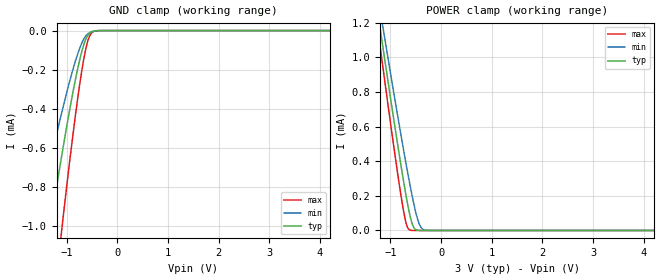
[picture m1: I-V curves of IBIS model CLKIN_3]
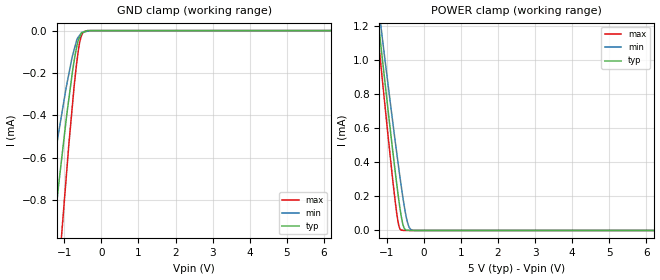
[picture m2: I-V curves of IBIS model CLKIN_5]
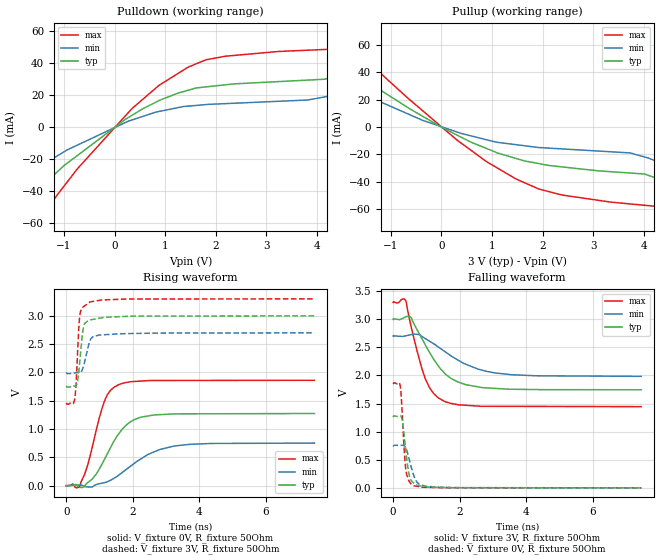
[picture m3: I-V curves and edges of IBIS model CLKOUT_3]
|Texas Instruments Incorporated
|Two 1-Bit, 10MHz, 2nd - Order Delta-Sigma Modulators
| Marketing part#   Digital Voltage Range   Package-type   #pins
|ADS1205IRGER   2.7V to 5.5V   QFN   24
|ADS1205IRGET   2.7V to 5.5V   QFN   24
|ADS1209SPW   2.7V to 5.5V   TSSOP   24
|ADS1209SPWR   2.7V to 5.5V   TSSOP   24
[IBIS Ver]   4.0
[File name]   ads1205_9.ibs
[File Rev]   1.0
[Date]   02/23/2010
[Source]   Texas Instruments Incorporated.
   Analog-eLab, HPA
   12500 TI Blvd
   Dallas, TX -75243
   For Support e-mail: elab_ibis@list.ti.com
[Notes]   Revision History:
   1.0: 02/23/2010
   - Initial version of the model
   - Initial Model generated from simulations in TIspiceD
   - Model names with a trailing _3 contains the model for
   3V [2.7V and 3.3V]. Model names with trailing _5 contains
   the model for 5V [4.5V and 5.5V] operation.
   - Model not matched to measurements
   - C_comp: Ignore warnings related to min and max values of
   ccomp. The device process of these products is CMOS. The
   ccomp values are based on PVT variations as seen in
   simulations
[Disclaimer]
 This product is designed as an aid for customers of Texas Instruments.
 No warranties, either expressed or implied, with respect to this third
 party software [if any] or with respect to its fitness for any
 particular purpose is claimed by Texas Instruments or the author. The
 software [if any] is provided solely on an "as is" basis. The entire
 risk as to its quality and performance is with the customer
[Copyright] [C] Copyright 2010 Texas Instruments Incorporated.
   All rights reserved.
|   ADS1205
[Component]   ADS1205rge
[Manufacturer] TI   |QFN package, 24-pin
[Package]
|variable   typ   min   max
R_pkg   0.041250   0.000780   0.051560
L_pkg   0.989262nH   0.176530nH   1.226320nH
C_pkg   0.170271pF   0.099550pF   0.190160pF
[Pin] signal_name  model_name  R_pin  L_pin C_pin
1   REFINB   TERM   0.04895  1.17050nH  0.16737pF
2   AGND   TERM   0.04084  0.96823nH  0.17417pF
3   AVDD   TERM   0.03902  0.92564nH  0.17135pF
4   AVDD   TERM   0.03955  0.93760nH  0.17281pF
5   AGND   TERM   0.04334  1.02645nH  0.18033pF
6   CLKSEL   CLKSEL   0.04571  1.09072nH  0.16450pF
7   CLKIN   CLKIN   0.04780  1.14015nH  0.16895pF
8   BVDD   POWER   0.04468  1.05593nH  0.18370pF
9   BGND   GND   0.04453  1.04910nH  0.18273pF
10   CLKOUT   CLKOUT   0.04778  1.12594nH  0.18715pF
11   OUTB   OUTB   0.05004  1.18148nH  0.19016pF
12   OUTA   OUTA   0.05156  1.22632nH  0.17289pF
13   AGND   TERM   0.04529  1.07336nH  0.16265pF
14   REFOUT   TERM   0.04455  1.04803nH  0.18209pF
15   AVDD   TERM   0.03980  0.93443nH  0.17351pF
16   AVDD   TERM   0.03902  0.91648nH  0.17120pF
17   AGND   TERM   0.04084  0.95994nH  0.17392pF
18   REFINA   TERM   0.04895  1.16087nH  0.16709pF
19   NC   NC   0.00078  0.17653nH  0.09956pF
20   CHA_P   TERM   0.04848  1.14386nH  0.18705pF
21   CHA_N   TERM   0.04462  1.05133nH  0.18325pF
22   CHB_N   TERM   0.04462  1.05344nH  0.18332pF
23   CHB_P   TERM   0.04848  1.14942nH  0.18720pF
24   NC   NC   0.00078  0.17653nH  0.09955pF
|   ADS1209
[Component]   ADS1209pw
[Manufacturer] TI   |TSSOP package, 24-pin
[Package]
|variable   typ   min   max
R_pkg  0.075590   0.004610   0.100660
L_pkg  2.215655nH 0.982720nH 3.019760nH
C_pkg  0.504497pF 0.380470pF 0.676480pF
[Pin] signal_name  model_name  R_pin  L_pin C_pin
1   AVDD   TERM   0.09322  2.96094nH  0.67218pF
2   AGND   TERM   0.09431  2.71108nH  0.58907pF
3   REFIN_A   TERM   0.09280  2.37002nH  0.49030pF
4   NC   TERM   0.00461  0.98272nH  0.38051pF
5   CHA_P   TERM   0.06838  1.90185nH  0.43543pF
6   CHA_N   TERM   0.06215  1.77364nH  0.41642pF
7   CHB_N   TERM   0.06215  1.77570nH  0.41648pF
8   CHB_P   TERM   0.06838  1.90665nH  0.43554pF
9   NC   TERM   0.00461  0.98278nH  0.38047pF
10   REFIN_B   TERM   0.09280  2.37806nH  0.49045pF
11   AGND   TERM   0.09431  2.71966nH  0.58921pF
12   AVDD   TERM   0.09328  2.97677nH  0.67017pF
13   AVDD   TERM   0.09564  3.01282nH  0.67576pF
14   AGND   TERM   0.09869  2.79683nH  0.59712pF
15   CLKSEL   CLKSEL   0.09186  2.35943nH  0.49325pF
16   CLKIN   CLKIN   0.07009  1.95030nH  0.44921pF
17   BVDD   POWER   0.06237  1.79861nH  0.43126pF
18   BGND   GND   0.06132  1.75914nH  0.41532pF
19   CLKOUT   CLKOUT   0.06753  1.86708nH  0.42092pF
20   OUTB   OUTB   0.07091  1.94594nH  0.43825pF
21   OUTA   OUTA   0.07669  2.06216nH  0.45415pF
22   AGND   TERM   0.09104  2.33841nH  0.49101pF
23   REFOUT   TERM   0.10066  2.82536nH  0.59897pF
24   AVDD   TERM   0.09636  3.01976nH  0.67648pF
|   Model Selectors
[Model Selector]  CLKIN
CLKIN_3   3V digital input
CLKIN_5   5V digital input
[Model Selector]  CLKSEL
CLKSEL_3  3V digital input
CLKSEL_5  5V digital input
[Model Selector]  CLKOUT
CLKOUT_3   3V digital output
CLKOUT_5   5V digital output
[Model Selector]  OUTA
OUTA_3   3V digital output
OUTA_5   5V digital output
[Model Selector]  OUTB
OUTB_3   3V digital output
OUTB_5   5V digital output
|   TERM Model
[Model] TERM
Model_type Terminator
C_comp   0   0   0
| variable   typ   min   max
[Voltage Range]   3.0V   2.7V   5.5V
[GND Clamp Reference]   0V   0V   0V
|Operating Temperature
[Temperature Range]   27   105   -40
| Models and submodels in the file (11): TERM (Terminator), CLKIN_3 (Input), CLKIN_5 (Input), CLKSEL_3 (Input), CLKSEL_5 (Input), CLKOUT_3 (Output), CLKOUT_5 (Output), OUTA_3 (Output), OUTA_5 (Output), OUTB_3 (Output), OUTB_5 (Output)
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|   CLKIN INPUT 3V Model
[Model] CLKIN_3
Model_type Input
| Signals  CKLIN
Vinl = 800.000mV
Vinh = 2.000V
|   typ   min   max
C_comp   5.7368190e-13   6.3979300e-13   5.1832840e-13
[Voltage Range]   3.000V   2.70V   3.60V
[Temperature Range]   27.0   105.0   -40.0
[GND Clamp Reference]   0V   0V   0V
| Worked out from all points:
|   GND clamp passes 1 mA (typ) near -1.32 V on its own axis
|   POWER clamp passes 1 mA (typ) near -1.12 V on its own axis
[GND Clamp]
|   Voltage   I[typ]   I[min]   I[max]
-3V       -4.625mA   -3.037mA   -7.229mA
-1.625V   -1.519mA   -1.024mA   -2.313mA
-1.333V   -1.02mA    -681.2uA   -1.582mA
-1.116V   -670uA     -440.6uA   -1.065mA
-1.059V   -580.8uA   -379.4uA   -931.7uA
-876.1mV  -316.1uA   -199.3uA   -533.8uA
-722.1mV  -128.1uA   -77.05uA   -240.3uA
-613.1mV  -39.28uA   -25.08uA   -83.29uA
-577mV    -22.76uA   -15.96uA   -48.79uA
-519.5mV  -8.31uA    -7.542uA   -16.38uA
-362.3mV  -136.9nA   -672.6nA   -110.2nA
5.991V    0A         0A         0A
[POWER Clamp]
|   Voltage   I[typ]   I[min]   I[max]
-3V       4.815mA    4.568mA    5.078mA
-1.317V   1.394mA    1.478mA    1.312mA
-1.221V   1.204mA    1.306mA    1.102mA
-1.196V   1.154mA    1.26mA     1.047mA
-1.129V   1.022mA    1.141mA    901.9uA
-772.7mV  342.4uA    520.1uA    168uA
-686.6mV  194.4uA    378.1uA    39.04uA
-615.2mV  88.7uA     265.8uA    2.489uA
-532.6mV  14.55uA    147uA      34.23nA
-440.5mV  528.1nA    45.68uA    118.1fA
-301.9mV  206.5pA    1.337uA    0A
5.991V    0A         0A         0A
|   CLKIN INPUT 5V Model
[Model] CLKIN_5
Model_type Input
| Signals   CLKIN
Vinl = 1.65V
Vinh = 3.15V
| variable   typ   min   max
C_comp   5.1340260e-13   5.5562810e-13   4.7532860e-13
[Voltage Range]   5   4.5   5.5
[Temperature Range]   27   105   -40
[GND Clamp Reference]   0   0   0
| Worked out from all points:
|   GND clamp passes 1 mA (typ) near -1.32 V on its own axis
|   POWER clamp passes 1 mA (typ) near -1.12 V on its own axis
[GND Clamp]
|   Voltage   I(typ)   I(min)   I(max)
-5V       -11.05mA   -7.434mA   -16.78mA
-1.642V   -1.552mA   -1.048mA   -2.356mA
-1.496V   -1.299mA   -871.9uA   -1.987mA
-1.282V   -937.7uA   -625.1uA   -1.458mA
-1.065V   -594.5uA   -388.9uA   -946.9uA
-868.6mV  -309.9uA   -196uA     -518.2uA
-764.7mV  -175uA     -109.6uA   -319.2uA
-671.6mV  -82.15uA   -48.87uA   -159.8uA
-607.5mV  -39.56uA   -27.19uA   -77.22uA
-558.7mV  -20.55uA   -15.56uA   -35.54uA
-461.7mV  -6.059uA   -6.081uA   -4.051uA
9.985V    0A         0A         0A
[POWER Clamp]
|   Voltage   I(typ)   I(min)   I(max)
-5V       8.926mA    8.285mA    9.599mA
-1.254V   1.269mA    1.364mA    1.174mA
-1.208V   1.178mA    1.282mA    1.074mA
-1.126V   1.016mA    1.136mA    895.5uA
-780.8mV  357.6uA    534uA      182.6uA
-683.3mV  189.1uA    373.3uA    35.65uA
-607.5mV  79.63uA    254.7uA    1.713uA
-533.8mV  15.09uA    149.1uA    212.2nA
-434.3mV  1.46uA     40.92uA    13.13nA
-370.2mV  38.02nA    9.541uA    13.05nA
-294.8mV  37.74nA    1.072uA    12.96nA
9.985V    0A         0A         0A
|   CLKOUT OUTPUT 3V Model
[Model] CLKOUT_3
Model_type Output
|Signal CLKOUT
Polarity   Non-Inverting
Enable   Active-Low
Vmeas = 1.5
Vref = 1.5
Cref = 15pF
Rref = 50
|   typ   min   max
|   AVERAGE
C_comp   2.2907165e-12   2.3755725e-12   2.2317525e-12
|   OUTPUT HIGH
|C_comp   2.6042970e-12   2.6735910e-12   2.5815490e-12
|   OUTPUT LOW
|C_comp   1.9771360e-12   2.0775540e-12   1.8819560e-12
[Voltage Range]   3   2.7   3.3
[Temperature Range]   27   105   -40
[Pullup Reference]   3   2.7   3.3
[Pulldown Reference]   0   0   0
[Power Clamp Reference]   3   2.7   3.3
[GND Clamp Reference]   0   0   0
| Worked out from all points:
|   slope of the pulldown table from 0 to 0.45 V, typ, clamps not added: 46.7 ohm
|   slope of the pullup table from 0 to 0.45 V, typ, clamps not added: 52.7 ohm
|   falling waveform, V_fixture 3V, R_fixture 50Ohm: 20-80 % time 853ps typ, 1.25ns min, 550ps max; typ from 3 V to 1.74 V
|   rising waveform, V_fixture 0V, R_fixture 50Ohm: 20-80 % time 765ps typ, 1.17ns min, 499ps max; typ from 0 V to 1.27 V
|   rising waveform, V_fixture 3V, R_fixture 50Ohm: 20-80 % time 131ps typ, 184ps min, 96.7ps max; typ from 1.74 V to 3 V
|   falling waveform, V_fixture 0V, R_fixture 50Ohm: 20-80 % time 159ps typ, 224ps min, 116ps max; typ from 1.27 V to 0 V
[Pulldown]
|   Voltage   I  typ   I  min   I  max
-3V       -128.9mA   -72.63mA   -232.6mA
-2.138V   -63.78mA   -40.45mA   -101.5mA
-1.562V   -40.62mA   -26.21mA   -62.54mA
-735.8mV  -17.77mA   -11.27mA   -26.09mA
338.9mV   7.199mA    4.368mA    11.31mA
1.481V    23.18mA    13.13mA    37.71mA
3.82V     29.28mA    16.87mA    47.92mA
4.671V    34.09mA    23.27mA    51.3mA
4.921V    38.26mA    32.68mA    54.63mA
5.232V    60.41mA    49.4mA     68.78mA
5.443V    79.74mA    61.23mA    99.82mA
5.991V    131.4mA    91.91mA    187.3mA
[Pullup]
|   Voltage   I  typ   I  min   I  max
-3V       132.9mA    76.01mA    237.1mA
-2.371V   74.24mA    43.33mA    136.6mA
-2.177V   58.35mA    37.7mA     105.8mA
-1.943V   48.03mA    32.4mA     72.89mA
-1.553V   35.35mA    24.09mA    51.25mA
302.6mV   -5.749mA   -3.526mA   -9.31mA
1.917V    -26.68mA   -14.97mA   -45.23mA
4.105V    -35.55mA   -22.84mA   -57.64mA
4.927V    -52.46mA   -37.34mA   -75.92mA
5.368V    -72.73mA   -54.77mA   -96.79mA
5.585V    -91.3mA    -66.05mA   -122.1mA
5.991V    -128mA     -87.92mA   -185mA
[Ramp]
R_load = 50
|   typ   min   max
dV/dt_r   0.764987/7.60195e-10   0.451646/1.14876e-09   1.11746/4.98193e-10
dV/dt_f   0.753304/8.48045e-10   0.430363/1.24194e-09   1.11358/5.48131e-10
[Falling Waveform]
V_fixture = 3V
V_fixture_min = 2.7V
V_fixture_max = 3.3V
R_fixture = 50Ohm
C_fixture = 0F
|   Time   V  typ   V  min   V  max
0s        3V         2.7V       3.3V
375.4ps   3.039V     2.703V     3.333V
543.8ps   3.029V     2.726V     2.859V
733.8ps   2.796V     2.729V     2.402V
966.2ps   2.545V     2.656V     1.943V
1.218ns   2.287V     2.562V     1.679V
1.542ns   2.042V     2.429V     1.539V
2.161ns   1.839V     2.204V     1.469V
3.091ns   1.768V     2.042V     1.45V
7.457ns   1.744V     1.983V     1.444V
[Rising Waveform]
V_fixture = 0V
V_fixture_min = 0V
V_fixture_max = 0V
R_fixture = 50Ohm
C_fixture = 0F
|   Time   V  typ   V  min   V  max
0s        798.5pV    4.863nV    672.5pV
414.5ps   -29.97mV   13.44mV    -258.3uV
643.5ps   55.44mV    -20.82mV   363.2mV
906.6ps   209.5mV    20.46mV    993.4mV
1.15ns    468mV      54.87mV    1.496V
1.324ns   664.7mV    94.39mV    1.68V
1.568ns   909.2mV    183.1mV    1.783V
2.213ns   1.205V     462.7mV    1.847V
3.222ns   1.268V     698.1mV    1.859V
7.457ns   1.275V     752.7mV    1.862V
[Rising Waveform]
V_fixture = 3V
V_fixture_min = 2.7V
V_fixture_max = 3.3V
R_fixture = 50Ohm
C_fixture = 0F
|   Time   V  typ   V  min   V  max
0s        1.744V     1.982V     1.444V
243.2ps   1.759V     1.99V      1.501V
292.8ps   1.762V     1.996V     1.767V
341.9ps   1.857V     2V         2.368V
385ps     2.063V     1.994V     2.857V
415.4ps   2.252V     1.996V     3.04V
520.2ps   2.803V     2.115V     3.162V
712.2ps   2.925V     2.559V     3.244V
1.601ns   2.985V     2.683V     3.292V
7.457ns   3V         2.7V       3.3V
[Falling Waveform]
|Gnd
V_fixture = 0V
V_fixture_min = 0V
V_fixture_max = 0V
R_fixture = 50Ohm
C_fixture = 0F
|   Time   V  typ   V  min   V  max
0s        1.275V     752.8mV    1.862V
209.5ps   1.277V     756.6mV    1.824V
277.1ps   1.197V     756.5mV    1.284V
338.9ps   898.3mV    747.1mV    622.7mV
383ps     655.8mV    709.6mV    325.5mV
489.3ps   216.5mV    495.3mV    109.8mV
617.6ps   86.63mV    224.5mV    38.3mV
781ps     33.55mV    65.53mV    20.58mV
1.28ns    8.672mV    11.82mV    4.993mV
7.457ns   46.03nV    3.895uV    -514.7pV
